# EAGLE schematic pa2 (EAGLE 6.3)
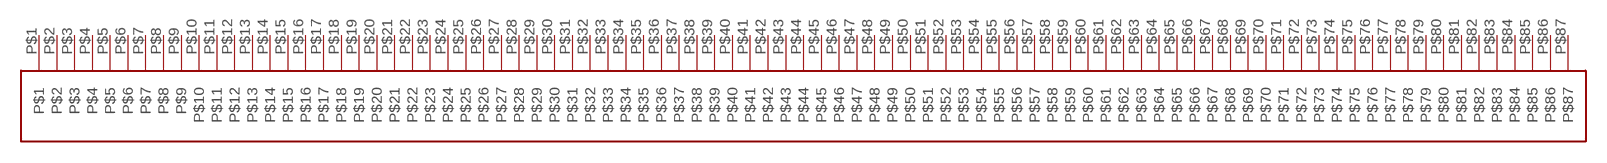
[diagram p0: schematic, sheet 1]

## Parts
U$1  PA2  [PA2]
Unconnected: U$1.P$1 U$1.P$2 U$1.P$3 U$1.P$4 U$1.P$5 U$1.P$6 U$1.P$7 U$1.P$8 U$1.P$9 U$1.P$10 U$1.P$11 U$1.P$12 U$1.P$13 U$1.P$14 U$1.P$15 U$1.P$16 U$1.P$17 U$1.P$18 U$1.P$19 U$1.P$20 U$1.P$21 U$1.P$22 U$1.P$23 U$1.P$24 U$1.P$25 U$1.P$26 U$1.P$27 U$1.P$28 U$1.P$29 U$1.P$30 U$1.P$31 U$1.P$32 U$1.P$33 U$1.P$34 U$1.P$35 U$1.P$36 U$1.P$37 U$1.P$38 U$1.P$39 U$1.P$40 U$1.P$41 U$1.P$42 U$1.P$43 U$1.P$44 U$1.P$45 U$1.P$46 U$1.P$47 U$1.P$48 U$1.P$49 U$1.P$50 U$1.P$51 U$1.P$52 U$1.P$53 U$1.P$54 U$1.P$55 U$1.P$56 U$1.P$57 U$1.P$58 U$1.P$59 U$1.P$60 U$1.P$61 U$1.P$62 U$1.P$63 U$1.P$64 U$1.P$65 U$1.P$66 U$1.P$67 U$1.P$68 U$1.P$69 U$1.P$70 U$1.P$71 U$1.P$72 U$1.P$73 U$1.P$74 U$1.P$75 U$1.P$76 U$1.P$77 U$1.P$78 U$1.P$79 U$1.P$80 U$1.P$81 U$1.P$82 U$1.P$83 U$1.P$84 U$1.P$85 U$1.P$86 U$1.P$87

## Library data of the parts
U$1 = FE-I4:PA2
